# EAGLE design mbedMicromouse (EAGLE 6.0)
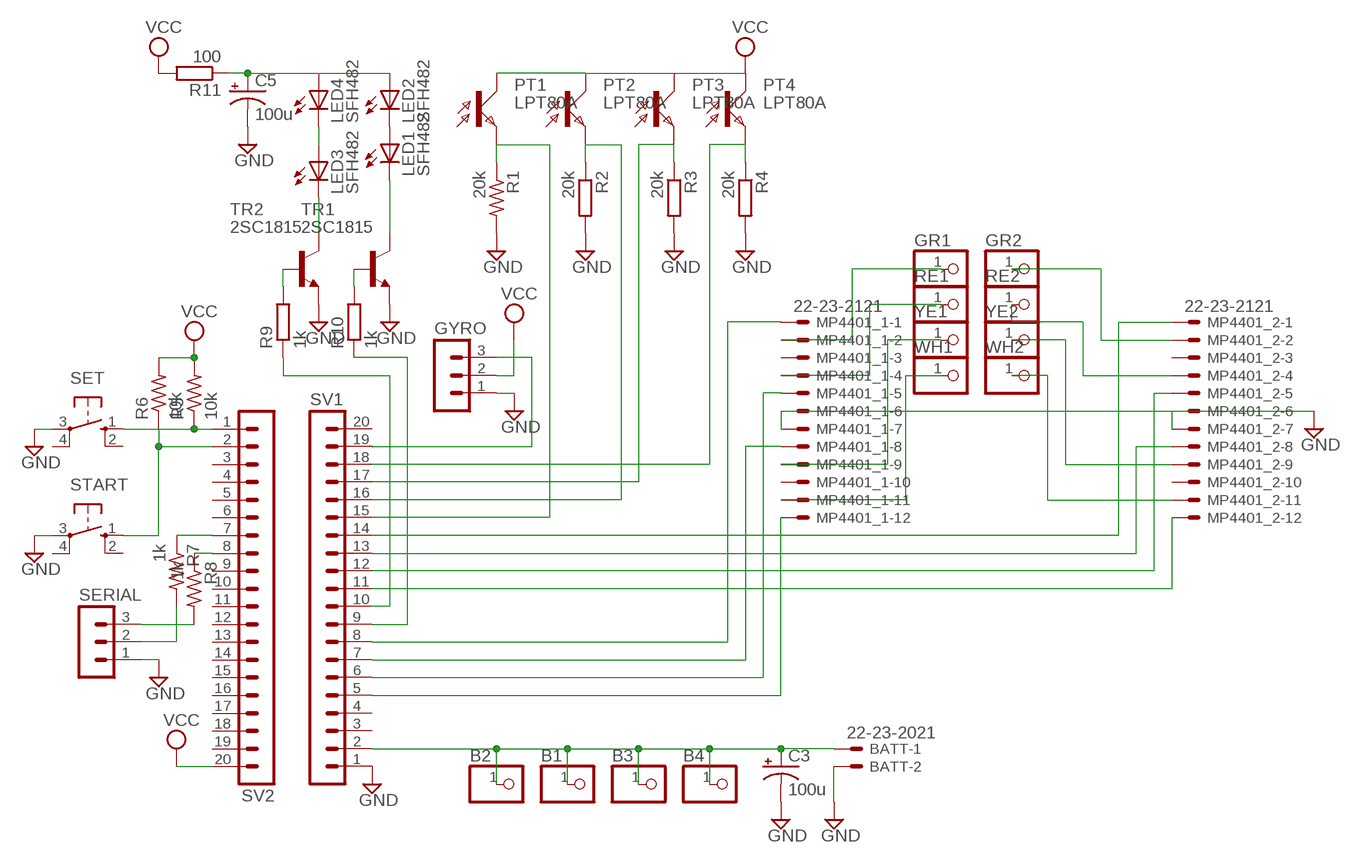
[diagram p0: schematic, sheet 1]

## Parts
B1  PINHD-1X1  [1X01]
B2  PINHD-1X1  [1X01]
B3  PINHD-1X1  [1X01]
B4  PINHD-1X1  [1X01]
BATT  22-23-2021  [22-23-2021]
C3  100u  CPOL-USTT2D5  [TT2D5]
C5  100u  CPOL-USTT2D5  [TT2D5]
GR1  PINHD-1X1  [1X01]
GR2  PINHD-1X1  [1X01]
GYRO  MA03-1  [MA03-1]
LED1  SFH482  [SFH482]
LED2  SFH482  [SFH482]
LED3  SFH482  [SFH482]
LED4  SFH482  [SFH482]
MP4401_1  22-23-2121  [22-23-2121]
MP4401_2  22-23-2121  [22-23-2121]
PT1  LPT80A  [LPT80A]
PT2  LPT80A  [LPT80A]
PT3  LPT80A  [LPT80A]
PT4  LPT80A  [LPT80A]
R1  20k  R-US_0204/2V  [0204V]
R2  20k  R-EU_0204/2V  [0204V]
R3  20k  R-EU_0204/2V  [0204V]
R4  20k  R-EU_0204/2V  [0204V]
R5  10k  R-US_0204/2V  [0204V]
R6  10k  R-US_0204/2V  [0204V]
R7  1k  R-US_0204/2V  [0204V]
R8  1k  R-US_0204/2V  [0204V]
R9  1k  R-EU_0204/2V  [0204V]
R10  1k  R-EU_0204/2V  [0204V]
R11  100  R-EU_0204/2V  [0204V]
RE1  PINHD-1X1  [1X01]
RE2  PINHD-1X1  [1X01]
SERIAL  MA03-1  [MA03-1]
SET  10-XX  [B3F-10XX]
START  10-XX  [B3F-10XX]
SV1  MA20-1  [MA20-1]
SV2  MA20-1  [MA20-1]
TR1  2SC1815  [TO92-ECB]
TR2  2SC1815  [TO92-ECB]
WH1  PINHD-1X1  [1X01]
WH2  PINHD-1X1  [1X01]
YE1  PINHD-1X1  [1X01]
YE2  PINHD-1X1  [1X01]

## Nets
GND: BATT.2 C3.- C5.- GYRO.1 MP4401_1.6 MP4401_1.7 MP4401_2.6 MP4401_2.7 R1.2 R2.2 R3.2 R4.2 SERIAL.1 SET.3(P) START.3(P) SV1.1 TR1.E TR2.E
N$1: PT3.E R3.1 SV1.17
N$2: R10.2 TR1.B
N$3: MP4401_1.1 SV1.8
N$4: R5.1 SET.1(S) SV2.1
N$5: R6.1 START.1(S) SV2.2
N$6: GYRO.3 SV1.19
N$7: PT4.E R4.1 SV1.18
N$8: PT2.E R2.1 SV1.16
N$9: R7.1 SV2.7
N$10: R8.2 SERIAL.3
N$11: C5.+ LED2.A LED4.A R11.1
N$12: LED3.A LED4.K(C)
N$13: R7.2 SERIAL.2
N$14: LED1.A LED2.K(C)
N$15: R8.1 SV2.8
N$16: MP4401_2.12 SV1.11
N$17: MP4401_1.5 SV1.6
N$18: LED3.K(C) TR2.C
N$19: R9.2 TR2.B
N$21: LED1.K(C) TR1.C
N$22: R10.1 SV1.9
N$25: B1.1 B2.1 B3.1 B4.1 BATT.1 C3.+ SV1.2
N$27: PT1.E R1.1 SV1.15
N$28: MP4401_2.1 SV1.14
N$29: R9.1 SV1.10
N$39: MP4401_1.8 SV1.7
N$41: MP4401_2.5 SV1.12
N$44: GR1.1 MP4401_1.2
N$45: MP4401_1.4 RE1.1
N$46: MP4401_1.11 WH1.1
N$47: MP4401_1.12 SV1.5
N$48: GR2.1 MP4401_2.2
N$49: MP4401_2.4 RE2.1
N$50: MP4401_2.9 YE2.1
N$51: MP4401_2.11 WH2.1
N$52: MP4401_1.9 YE1.1
N$61: MP4401_2.8 SV1.13
VCC: GYRO.2 PT1.C PT2.C PT3.C PT4.C R5.2 R6.2 R11.2 SV2.20
Unconnected: MP4401_1.3 MP4401_1.10 MP4401_2.3 MP4401_2.10 SET.2(S1) SET.4(P1) START.2(S1) START.4(P1) SV1.3 SV1.4 SV1.20 SV2.3 SV2.4 SV2.5 SV2.6 SV2.9 SV2.10 SV2.11 SV2.12 SV2.13 SV2.14 SV2.15 SV2.16 SV2.17 SV2.18 SV2.19

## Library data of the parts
B1-B4 GR1 GR2 RE1 RE2 WH1 WH2 YE1 YE2 = pinhead:PINHD-1X1: PIN HEADER
BATT = con-molex:22-23-2021: .100" (2.54mm) Center Header - 2 Pin
C3 C5 = resistor:CPOL-US: POLARIZED CAPACITOR, American symbol
GYRO SERIAL = con-lstb:MA03-1: PIN HEADER
LED1-LED4 = led:SFH482: IR LED
MP4401_1 MP4401_2 = con-molex:22-23-2121: .100" (2.54mm) Center Header - 12 Pin
PT1-PT4 = opto-trans-siemens:LPT80A: PHOTO TRANSISTOR
R1 R5-R8 = resistor:R-US_: RESISTOR, American symbol
R2-R4 R9 R10 = rcl:R-EU_: RESISTOR, European symbol
R11 = resistor:R-EU_: RESISTOR, European symbol
SET START = switch-omron:10-XX: OMRON SWITCH
SV1 SV2 = con-lstb:MA20-1: PIN HEADER; OC_FARNELL: unknown; OC_NEWARK: unknown
TR1 TR2 = transistor:2SC1815: NPN EPITAXIAL TRANSISTOR Source: TOSHIBA .. 2SC1815 1.pdf

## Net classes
1 +5V: width 0.61 mm, drill 0.406 mm
2 GND: width 0.914 mm, drill 0.406 mm

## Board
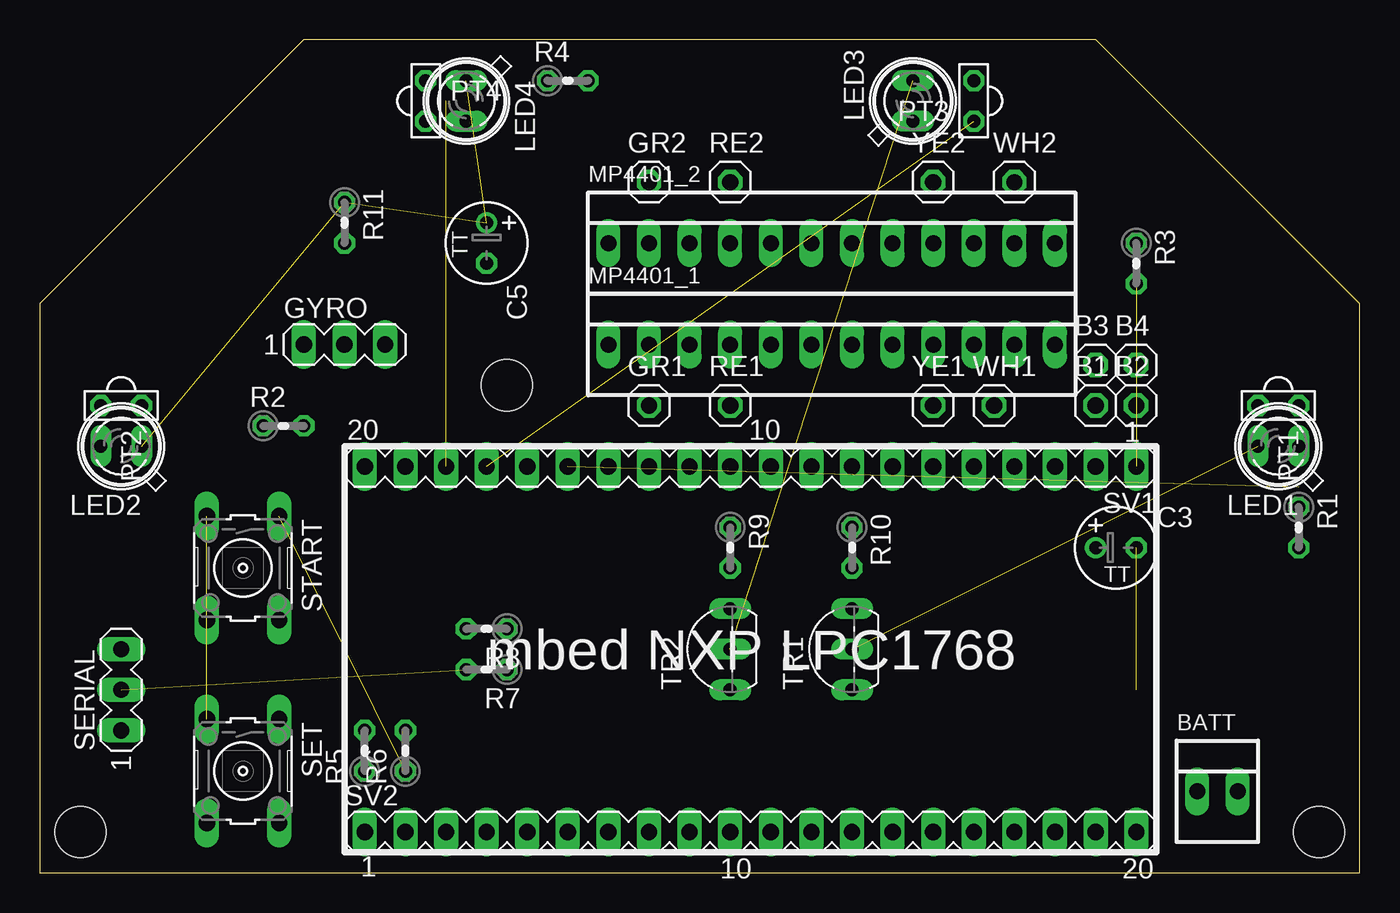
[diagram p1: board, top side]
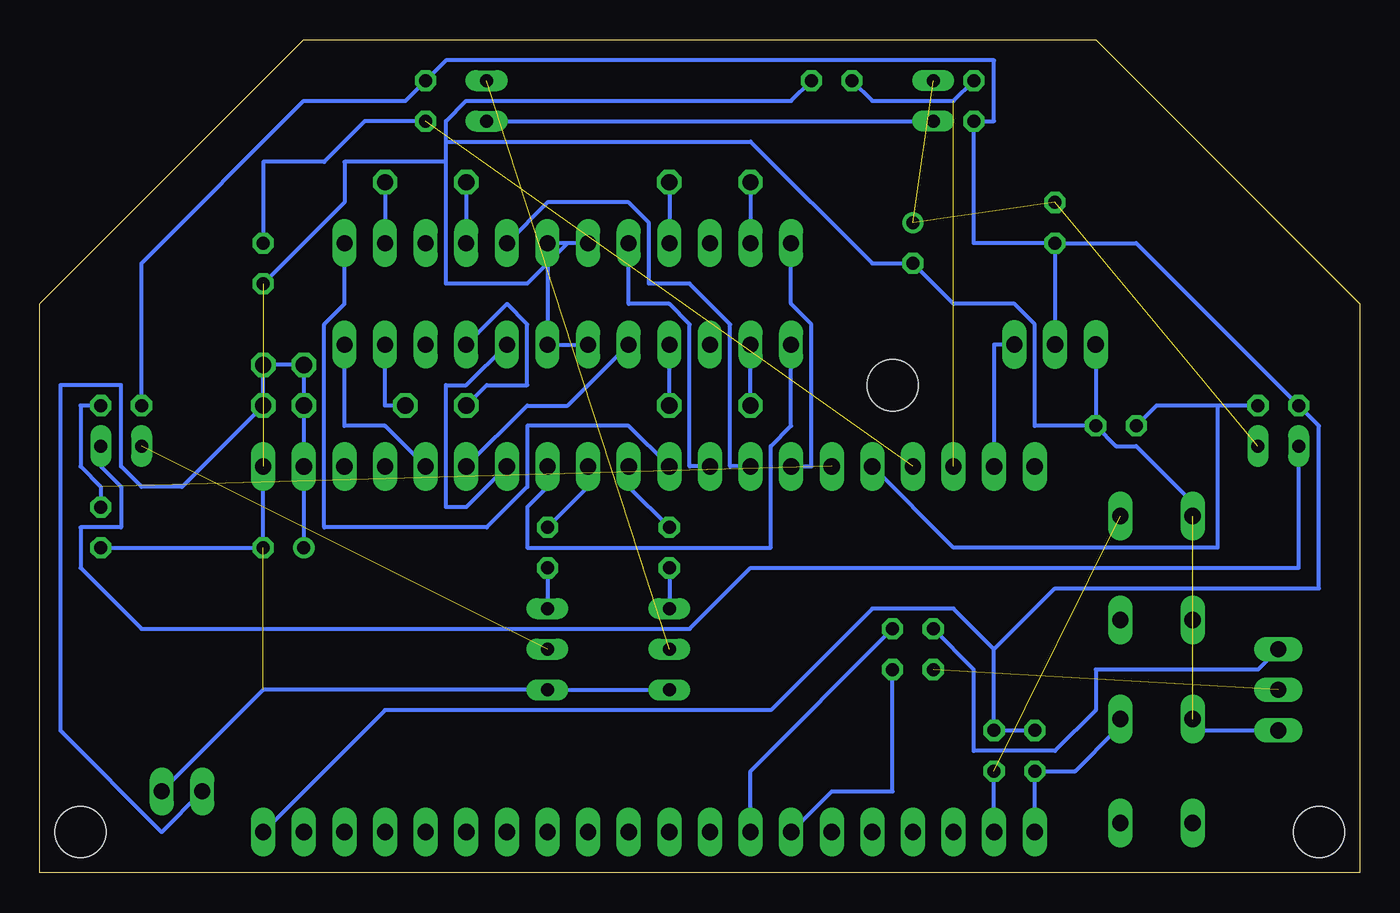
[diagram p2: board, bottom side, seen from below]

Size 82.55 x 52.07 mm. Coordinates in mm from the lower left corner, seen from the top.
Outline: 0,0 82.55,0 82.55,35.56 66.04,52.07 16.51,52.07 0,35.56 0,0
Copper layers (1*16): Top 0.035mm / dielectric 1.5mm / Bottom 0.035mm
Design rules: minimum track width 10mil, minimum drill 24mil, track to track 8mil, track to pad 8mil, pad to pad 8mil, via to via 8mil, smd to smd 8mil, copper to edge 40mil, drill to drill 8mil, minimum pad ring 10mil, minimum via ring 8mil, stop-mask expansion 4mil, vias tented up to drill 0mil, thermal gap 10mil
Holes 3.2 mm at 29.21,30.48 2.54,2.54 80.01,2.54

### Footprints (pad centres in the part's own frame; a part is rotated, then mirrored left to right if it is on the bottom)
1X01 = drill 1.016 octagon: 1 0,0
22-23-2021 = drill 1 long: 1 -1.27,0; 2 1.27,0
TT2D5 = drill 0.813: + -1.27,0 | drill 0.813 octagon: - 1.27,0
MA03-1 = drill 1.016 long: 1 -2.54,0; 2 0,0; 3 2.54,0
SFH482 = drill 0.813 long: A -1.27,0; K 1.27,0
22-23-2121 = drill 1 long: 1 -13.97,0; 2 -11.43,0; 3 -8.89,0; 4 -6.35,0; 5 -3.81,0; 6 -1.27,0; 7 1.27,0; 8 3.81,0; 9 6.35,0; 10 8.89,0; 11 11.43,0; 12 13.97,0
LPT80A = drill 0.813 octagon: C 0,-1.27; E 0,1.27
0204V = drill 0.813 octagon: 1 -1.27,0; 2 1.27,0
B3F-10XX = drill 1.016 long: 1 -3.251,2.261; 2 3.251,2.261; 3 -3.251,-2.261; 4 3.251,-2.261
MA20-1 = drill 1.016 long: 1 -24.13,0; 2 -21.59,0; 3 -19.05,0; 4 -16.51,0; 5 -13.97,0; 6 -11.43,0; 7 -8.89,0; 8 -6.35,0; 9 -3.81,0; 10 -1.27,0; 11 1.27,0; 12 3.81,0; 13 6.35,0; 14 8.89,0; 15 11.43,0; 16 13.97,0; 17 16.51,0; 18 19.05,0; 19 21.59,0; 20 24.13,0
TO92-ECB = drill 0.813 long: B 2.54,0; C 0,0; E -2.54,0

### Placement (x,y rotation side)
B1  66.04,29.21 0 top
B2  68.58,29.21 0 top
B3  66.04,31.75 0 top
B4  68.58,31.75 0 top
BATT  73.66,5.08 0 top
C3  67.31,20.32 0 top
C5  27.94,39.37 270 top
GR1  38.1,29.21 0 top
GR2  38.1,43.18 0 top
GYRO  19.05,33.02 0 top
LED1  77.47,26.67 180 top
LED2  5.08,26.67 180 top
LED3  54.61,48.26 90 top
LED4  26.67,48.26 270 top
MP4401_1  49.53,33.02 0 top
MP4401_2  49.53,39.37 0 top
PT1  77.47,29.21 270 top
PT2  5.08,29.21 270 top
PT3  58.42,48.26 180 top
PT4  24.13,48.26 0 top
R1  78.74,21.59 270 top
R2  15.24,27.94 0 top
R3  68.58,38.1 270 top
R4  33.02,49.53 0 top
R5  20.32,7.62 90 top
R6  22.86,7.62 90 top
R7  27.94,12.7 180 top
R8  27.94,15.24 180 top
R9  43.18,20.32 270 top
R10  50.8,20.32 270 top
R11  19.05,40.64 270 top
RE1  43.18,29.21 0 top
RE2  43.18,43.18 0 top
SERIAL  5.08,11.43 90 top
SET  12.7,6.35 270 top
START  12.7,19.05 270 top
SV1  44.45,25.4 180 top
SV2  44.45,2.54 0 top
TR1  50.8,13.97 90 top
TR2  43.18,13.97 90 top
WH1  59.69,29.21 0 top
WH2  60.96,43.18 0 top
YE1  55.88,29.21 0 top
YE2  55.88,43.18 0 top

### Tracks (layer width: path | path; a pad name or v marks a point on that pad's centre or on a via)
GND  (3 unrouted)
  Bottom 0.254: GYRO.1 R2.2 | R2.2 20.32,27.94 20.32,34.29 21.59,35.56 25.4,35.56 C5.- 30.48,38.1 38.1,45.72 57.15,45.72 | R2.2 15.24,26.67 13.97,26.67 10.16,22.86 START.3 | MP4401_1.6 MP4401_1.7 50.8,38.1 | R4.2 35.56,48.26 55.88,48.26 57.15,46.99 57.15,45.72 | 57.15,44.45 57.15,36.83 52.07,36.83 50.8,38.1 | 57.15,44.45 57.15,45.72 | 49.53,39.37 50.8,38.1 | MP4401_2.6 49.53,39.37 | R3.2 63.5,41.91 63.5,44.45 57.15,44.45 | 49.53,39.37 MP4401_2.7 50.8,38.1 | SERIAL.1 10.16,8.89 SET.3 | TR2.E TR1.E 68.58,11.43 BATT.2 | R1.2 C3.- SV1.1
N$1  (1 unrouted)
  Bottom 0.254: R3.1 68.58,44.45 64.77,44.45 62.23,46.99 PT3.E
N$2
  Bottom 0.254: R10.2 TR1.B
N$3
  Bottom 0.254: MP4401_1.1 35.56,27.94 36.83,26.67 36.83,20.32 52.07,20.32 52.07,22.86 50.8,24.13 SV1.8
N$4
  Bottom 0.254: SV2.1 R5.1 17.78,6.35 15.24,8.89 SET.1
N$5  (1 unrouted)
  Bottom 0.254: SV2.2 R6.1
N$6
  Bottom 0.254: SV1.19 22.86,33.02 GYRO.3
N$7  (1 unrouted)
  Bottom 0.254: PT4.E 25.4,48.26 30.48,48.26 R4.1
N$8
  Bottom 0.254: R2.1 12.7,29.21 8.89,29.21 | PT2.E 8.89,29.21 | SV1.16 25.4,20.32 8.89,20.32 8.89,29.21
N$9
  Bottom 0.254: R7.1 29.21,5.08 33.02,5.08 SV2.7
N$10
  Bottom 0.254: R8.2 24.13,12.7 24.13,7.62 19.05,7.62 16.51,10.16 16.51,12.7 6.35,12.7 SERIAL.3
N$11  (3 unrouted)
N$12
  Bottom 0.254: LED3.A LED4.K
N$13  (1 unrouted)
N$14
  Bottom 0.254: LED2.K 3.81,19.05 38.1,19.05 41.91,15.24 76.2,15.24 80.01,19.05 80.01,21.59 77.47,21.59 77.47,24.13 78.74,25.4 LED1.A
N$15
  Bottom 0.254: R8.1 38.1,6.35 SV2.8
N$16
  Bottom 0.254: MP4401_2.12 63.5,35.56 64.77,34.29 64.77,21.59 54.61,21.59 52.07,24.13 52.07,27.94 45.72,27.94 SV1.11
N$17
  Bottom 0.254: MP4401_1.5 49.53,29.21 52.07,29.21 SV1.6
N$18  (1 unrouted)
N$19
  Bottom 0.254: R9.2 TR2.B
N$21  (1 unrouted)
N$22
  Bottom 0.254: R10.1 48.26,24.13 SV1.9
N$25
  Bottom 0.254: C3.+ SV1.2 B1.1 B3.1 B4.1 B2.1 73.66,24.13 76.2,24.13 77.47,25.4 77.47,30.48 81.28,30.48 81.28,8.89 74.93,2.54 BATT.1
N$27  (1 unrouted)
  Bottom 0.254: R1.1 78.74,24.13 80.01,25.4 80.01,29.21 PT1.E
N$28
  Bottom 0.254: MP4401_2.1 35.56,35.56 34.29,34.29 34.29,25.4 SV1.14
N$29
  Bottom 0.254: R9.1 45.72,24.13 SV1.10
N$39
  Bottom 0.254: MP4401_1.8 55.88,30.48 57.15,30.48 57.15,22.86 55.88,22.86 SV1.7
N$41
  Bottom 0.254: MP4401_2.5 45.72,35.56 43.18,35.56 41.91,34.29 41.91,25.4 SV1.12
N$44
  Bottom 0.254: GR1.1 MP4401_1.2
N$45
  Bottom 0.254: RE1.1 MP4401_1.4
N$46
  Bottom 0.254: MP4401_1.11 60.96,29.21 WH1.1
N$47
  Bottom 0.254: MP4401_1.12 63.5,27.94 60.96,27.94 SV1.5
N$48
  Bottom 0.254: GR2.1 MP4401_2.2
N$49
  Bottom 0.254: RE2.1 MP4401_2.4
N$50
  Bottom 0.254: YE2.1 MP4401_2.9
N$51
  Bottom 0.254: WH2.1 MP4401_2.11
N$52
  Bottom 0.254: MP4401_1.9 53.34,35.56 52.07,34.29 52.07,30.48 54.61,30.48 YE1.1
N$61
  Bottom 0.254: MP4401_2.8 50.8,41.91 45.72,41.91 44.45,40.64 44.45,36.83 41.91,36.83 39.37,34.29 39.37,25.4 SV1.13
VCC
  Bottom 0.254: PT1.C 76.2,38.1 66.04,48.26 59.69,48.26 PT3.C 57.15,50.8 22.86,50.8 22.86,46.99 PT4.C 24.13,39.37 R11.2 | R11.2 13.97,39.37 PT2.C 2.54,27.94 2.54,17.78 19.05,17.78 22.86,13.97 | R11.2 GYRO.2 | R5.2 R6.2 22.86,13.97 | SV2.20 60.96,10.16 36.83,10.16 30.48,16.51 25.4,16.51 22.86,13.97

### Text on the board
tNames: mbed NXP LPC1768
